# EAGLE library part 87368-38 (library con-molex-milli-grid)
RECEPTACAL
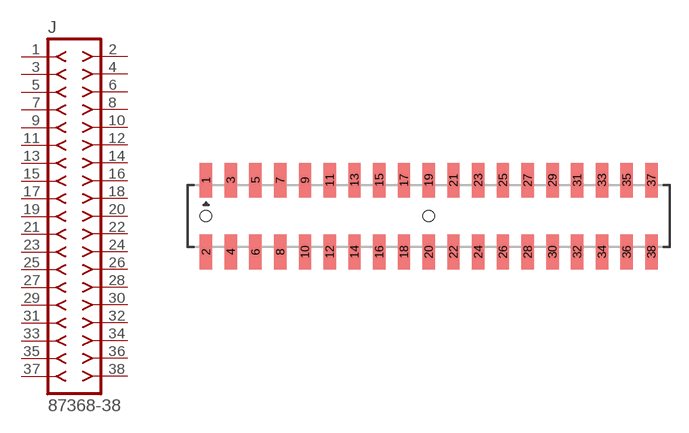
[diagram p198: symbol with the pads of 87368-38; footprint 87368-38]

Designator prefix J

## 87368-38  [87368-38]
1  1  pas
2  2  pas
3  3  pas
4  4  pas
5  5  pas
6  6  pas
7  7  pas
8  8  pas
9  9  pas
10  10  pas
11  11  pas
12  12  pas
13  13  pas
14  14  pas
15  15  pas
16  16  pas
17  17  pas
18  18  pas
19  19  pas
20  20  pas
21  21  pas
22  22  pas
23  23  pas
24  24  pas
25  25  pas
26  26  pas
27  27  pas
28  28  pas
29  29  pas
30  30  pas
31  31  pas
32  32  pas
33  33  pas
34  34  pas
35  35  pas
36  36  pas
37  37  pas
38  38  pas

## Footprint 87368-38 (pad centres in mm)
RECEPTACAL SMD Dual Row, Side Entry
smd 1 x 2.8: 1 -18,2.9; 2 -18,-2.9; 3 -16,2.9; 4 -16,-2.9; 5 -14,2.9; 6 -14,-2.9; 7 -12,2.9; 8 -12,-2.9; 9 -10,2.9; 10 -10,-2.9; 11 -8,2.9; 12 -8,-2.9; 13 -6,2.9; 14 -6,-2.9; 15 -4,2.9; 16 -4,-2.9; 17 -2,2.9; 18 -2,-2.9; 19 0,2.9; 20 0,-2.9; 21 2,2.9; 22 2,-2.9; 23 4,2.9; 24 4,-2.9; 25 6,2.9; 26 6,-2.9; 27 8,2.9; 28 8,-2.9; 29 10,2.9; 30 10,-2.9; 31 12,2.9; 32 12,-2.9; 33 14,2.9; 34 14,-2.9; 35 16,2.9; 36 16,-2.9; 37 18,2.9; 38 18,-2.9
hole 0.914 at -18,0
hole 0.914 at 0,0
